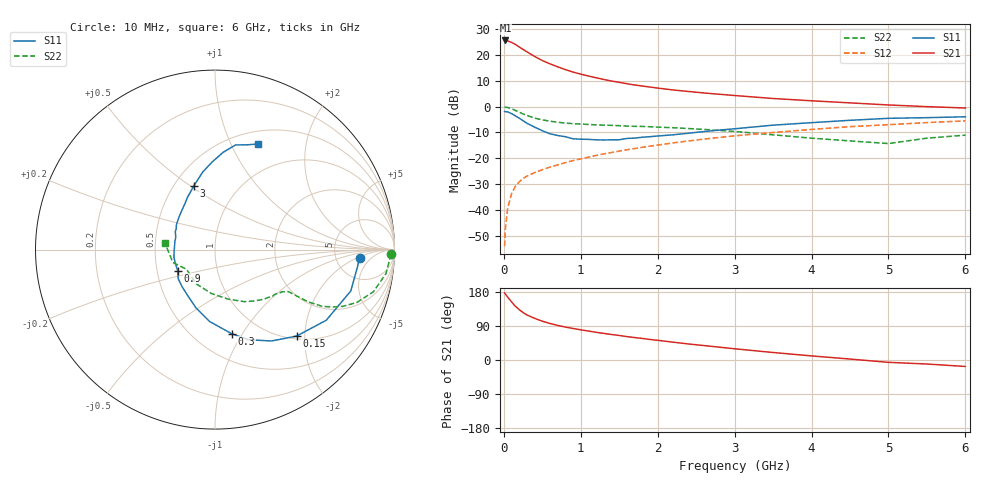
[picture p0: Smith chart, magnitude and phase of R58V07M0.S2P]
! SIEMENS Small Signal Semiconductors
! BFR183
! Si NPN RF Bipolar Junction Transistor in SOT23
! VCE = 8 V  IC = 7 mA
! Common Emitter S-Parameters:  May  1996
# GHz  S  MA  R  50
!  f  S11  S21  S12  S22
! GHz  MAG  ANG  MAG  ANG  MAG  ANG  MAG  ANG
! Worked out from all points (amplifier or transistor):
!   36 points, 10 MHz to 6 GHz, reference 50 ohm
!   highest |S21| = 25.6 dB at 20 MHz (marker M1)
!   |S21| within 3 dB of that: start of sweep to 225.2 MHz
!   unconditionally stable (mu >= 1): 945.5 MHz to 2.664 GHz
!   at 250 MHz: K = 0.50, MSG = 25.0 dB, |S12| = -27.8 dB
!   at 1.4 GHz: K = 1.05, MAG = 12.4 dB, |S12| = -17.8 dB
!   at 6 GHz: K = 0.88, MSG = 2.5 dB, |S12| = -5.5 dB
!   lowest NFmin = 1.25 dB at 450 MHz
!   S11 on the Smith chart (normalised r, x): 10 MHz: 8.69, -2.38; 150 MHz: 1.06, -1.82; 300 MHz: 0.74, -0.90; 900 MHz: 0.64, -0.16; 3 GHz: 0.63, +0.51; 6 GHz: 0.65, +1.28
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0.01  0.8067 -3.4  18.94 176.9  0.002 86.5  0.9832 -1.5
0.02  0.7995 -6.9  19.05 173.9  0.0044 84.2  0.9745 -3.2
0.05  0.791 -16.9  18.66 166.0  0.0109 80.8  0.9618 -8.0
0.1  0.7343 -32.4  17.43 153.6  0.0206 73.8  0.9134 -14.9
0.15  0.6622 -46.7  15.98 141.6  0.0288 68.6  0.8441 -20.4
0.2  0.5984 -58.3  14.27 133.0  0.0351 65.0  0.7803 -23.9
0.25  0.5355 -69.6  12.76 125.2  0.0408 62.0  0.7231 -26.3
0.3  0.4775 -78.8  11.48 118.9  0.0452 61.1  0.6741 -27.9
0.4  0.4016 -94.3  9.361 110.0  0.0529 59.9  0.6001 -29.2
0.5  0.3422 -107.9  7.792 102.4  0.0603 60.0  0.5541 -29.5
0.6  0.2983 -120.5  6.719 96.4  0.0677 59.9  0.5223 -29.6
0.7  0.2765 -131.5  5.886 91.3  0.0746 60.8  0.4989 -29.7
0.9  0.2386 -150.7  4.658 83.2  0.0905 61.4  0.4681 -29.9
1.1  0.2328 -169.2  3.91 76.4  0.1055 62.0  0.4519 -31.3
1.3  0.2262 175.3  3.348 70.2  0.1219 61.7  0.4384 -32.6
1.6  0.2426 155.7  2.773 61.7  0.1466 60.9  0.4205 -36.0
2.2  0.2852 130.6  2.101 47.1  0.1988 57.5  0.3903 -44.6
3  0.3729 108.6  1.64 29.6  0.2725 50.3  0.3317 -60.9
3.5  0.4382 98.9  1.436 19.8  0.3162 44.5  0.2851 -75.2
4.5  0.5441 85.2  1.182 2.5  0.41 33.0  0.2173 -118.8
5.5  0.6117 72.7  1 -10.6  0.4913 21.2  0.2455 -163.0
6  0.6361 67.7  0.94 -17.1  0.5303 13.5  0.2807 172.7
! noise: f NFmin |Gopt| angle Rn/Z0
0.45  1.25  0.18  42  0.22
0.9  1.3  0.22  110  0.2
1.8  2  0.33  180  0.14
